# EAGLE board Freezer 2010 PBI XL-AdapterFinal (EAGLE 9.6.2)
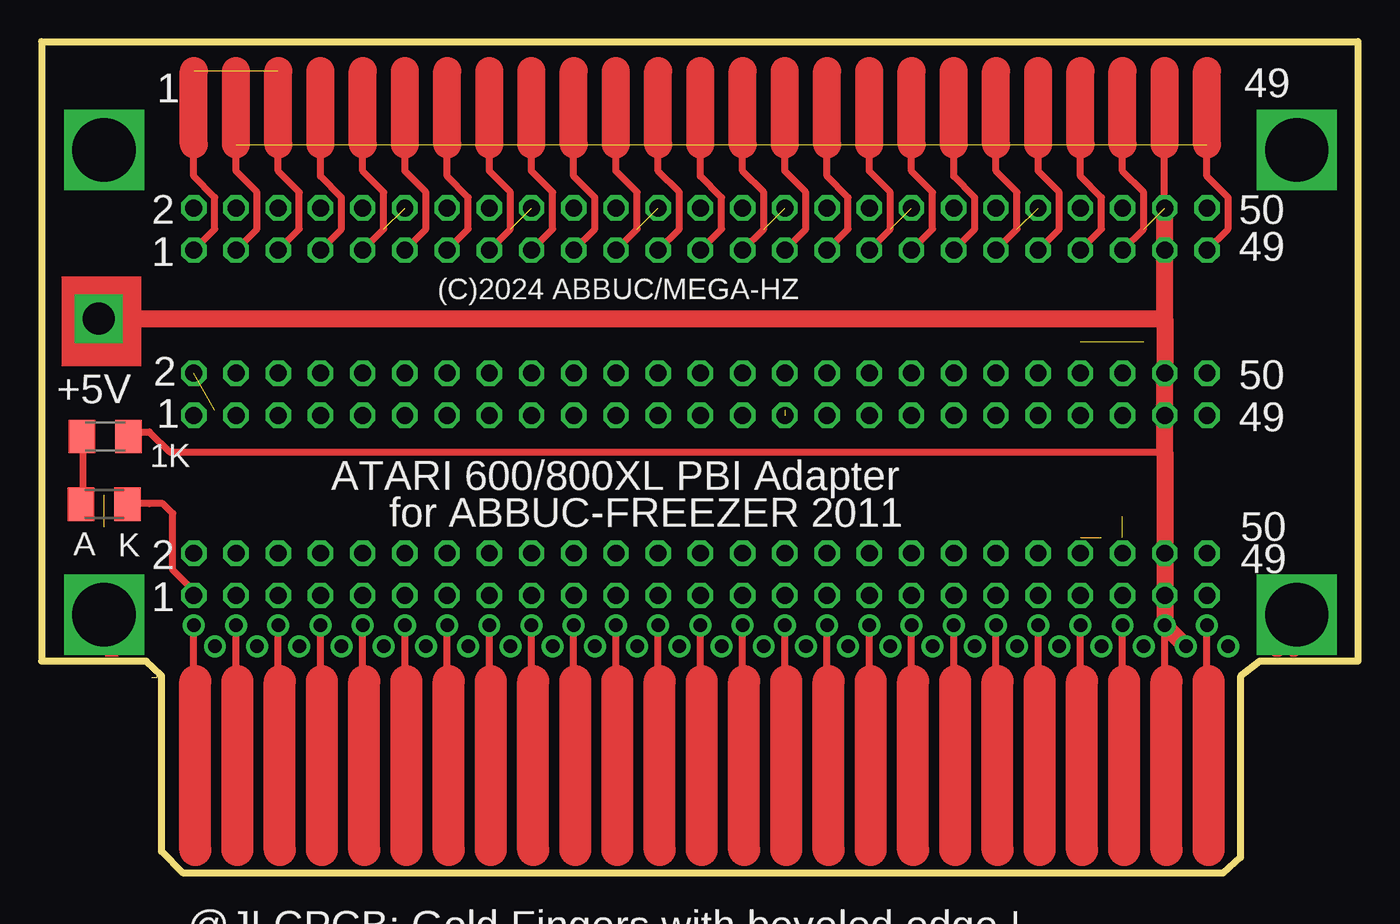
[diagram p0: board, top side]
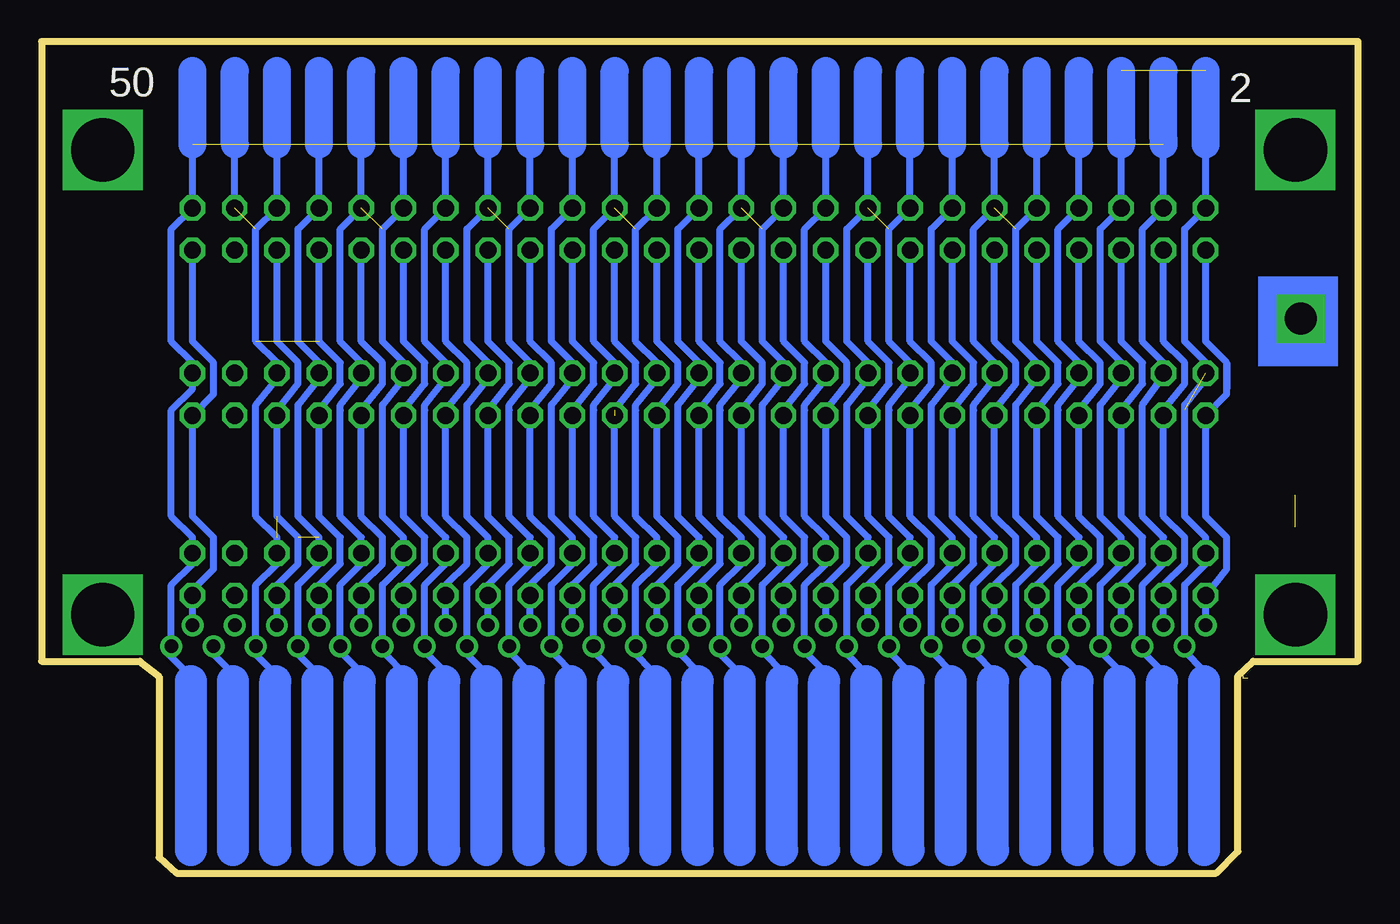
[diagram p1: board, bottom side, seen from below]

Size 79.2 x 50.05 mm. Coordinates in mm from the lower left corner, seen from the top.
Outline: 79.2,12.75 73.3,12.75 72.13,11.83 72.13,0.95 71.07,0 8.53,0 7.22,1.31 7.22,11.88 6.3,12.75 0,12.75 0,50.05 79.2,50.05 79.2,12.75
Copper layers (1*16): Top 0.035mm / dielectric 1.5mm / Bottom 0.035mm
Design rules "ITead_rule": minimum track width 6mil, minimum drill 12mil, track to track 6mil, track to pad 6mil, pad to pad 6mil, via to via 6mil, smd to smd 0mil, copper to edge 10mil, drill to drill 10mil, minimum pad ring 10mil, minimum via ring 6mil, stop-mask expansion 2mil, vias tented up to drill 100mil, thermal gap 10mil
Net classes: 2 3.3: width 0.508 mm, clearance 0.254 mm

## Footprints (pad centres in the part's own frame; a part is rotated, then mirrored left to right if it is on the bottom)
M1206 = smd 1.6 x 2: 1 -1.4,0; 2 1.4,0
XL-PBI = drill 0.813: A0 31.115,-8.255; A1 29.845,-6.985; A2 28.575,-8.255; A3 27.305,-6.985; A4 26.035,-8.255; A5 24.765,-6.985; A6 23.495,-8.255; A7 20.955,-8.255; A8 19.685,-6.985; A9 18.415,-8.255; A10 17.145,-6.985; A11 15.875,-8.255; A12 14.605,-6.985; A13 13.335,-8.255; A14 12.065,-6.985; A15 9.525,-6.985; AUDIO -27.305,-8.255; CAS -17.145,-8.255; D0 8.255,-8.255; D1 6.985,-6.985; D2 5.715,-8.255; D3 4.445,-6.985; D4 3.175,-8.255; D5 1.905,-6.985; D6 0.635,-8.255; D7 -0.635,-6.985; EXT.B -13.335,-6.985; EXTSEL 32.385,-6.985; GND -28.575,-6.985; GND2 -18.415,-6.985; GND3 -5.715,-6.985; GND4 -3.175,-6.985; GND5 22.225,-6.985; GND6 33.655,-8.255; GND7 10.795,-8.255; GND8 -1.905,-8.255; GND9 -22.225,-8.255; IRQ -9.525,-8.255; MPD -19.685,-8.255; NC2 -6.985,-8.255; NC3 -12.065,-8.255; NC4 -14.605,-8.255; PHI2 -4.445,-8.255; RAS -20.955,-6.985; RDY -10.795,-6.985; REF -15.875,-6.985; RST -8.255,-6.985; RW -23.495,-6.985; VCC -24.765,-8.255; VCC1 -26.035,-6.985

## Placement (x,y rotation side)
E$2  [M1206]  3.82,26.29 0 top
E$3  [M1206]  3.77,22.21 180 top
U$3  XL-PBI  [XL-PBI]  42.81,6.67 180 top

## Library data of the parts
E$2 E$3 = rcl
U$3 = wf-atari

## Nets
N$1: U$3.EXTSEL
N$16: U$3.AUDIO
N$28: U$3.VCC U$3.VCC1
N$32: U$3.GND9
N$33: U$3.MPD
N$34: U$3.CAS
N$35: U$3.NC4
N$37: U$3.NC3
N$38: U$3.IRQ
N$48: U$3.NC2
N$81: U$3.PHI2
N$88: U$3.GND8
N$89: U$3.D6
N$90: U$3.D4
N$91: U$3.D2
N$92: U$3.D0
N$93: U$3.GND7
N$94: U$3.A13
N$95: U$3.A11
N$96: U$3.A9
N$97: U$3.A7
N$98: U$3.A6
N$99: U$3.A4
N$102: U$3.RW
N$103: U$3.RAS
N$104: U$3.GND2
N$105: U$3.REF
N$106: U$3.EXT.B
N$107: U$3.RDY
N$108: U$3.RST
N$109: U$3.GND3
N$110: U$3.GND4
N$111: U$3.D7
N$112: U$3.D5
N$113: U$3.D3
N$114: U$3.D1
N$115: U$3.A15
N$116: U$3.A14
N$117: U$3.A12
N$118: U$3.A10
N$119: U$3.A8
N$120: U$3.GND5
N$122: U$3.A5
N$126: U$3.A1 U$3.A3
N$159: U$3.GND6
N$190: U$3.GND
N$307: U$3.A2
N$354: U$3.A0

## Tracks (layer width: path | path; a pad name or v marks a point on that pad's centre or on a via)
N$1  (via drill 1.02)  (1 unrouted)
  Bottom 0.406: 9.16,46.7 9.16,40.03 10.43,38.76 10.43,32 9.16,30.72 v9.16,30.09 | 10.43,27.87 10.43,21.48 9.16,20.21 v9.16,19.25 9.16,18.62 10.43,17.35 U$3.EXTSEL
N$16  (via drill 1.02)
  Bottom 0.406: U$3.AUDIO v70.12,16.72 70.12,17.03 68.85,18.3 68.85,20.21 70.12,21.48 70.12,27.55 68.85,28.82 68.85,30.72 70.12,32 v70.12,37.49
N$23  (via drill 1.02)
  other vias: 70.12,40.03
N$28  (via drill 1.02)
  Top 0.406: 4.78,26.56 6.49,26.56 7.7,25.35 67.58,25.35 67.6,25.35
  Top 1.016: 67.58,26.91 67.58,25.35 v67.58,19.25 v67.58,16.72 U$3.VCC U$3.VCC1
N$29  (via drill 1.02, 1.93)
  Top 0.406: 67.58,43.52 67.58,43.4 67.55,43.73 67.55,40.46 67.58,37.49
  Top 1.016: v67.58,27.55 v67.58,30.09 67.58,33.36 | 4.08,33.36 3.13,33.36 | 4.08,33.36 67.58,33.36 | v3.44,33.36 4.08,33.36 | 67.58,33.36 67.58,37.49 v67.58,40.03
N$30  (via drill 1.02)
  other vias: 65.04,40.03
N$31  (via drill 1.02)
  other vias: 62.5,40.03
N$32  (via drill 1.02)
  Bottom 0.406: U$3.GND9 v65.04,16.72
N$33  (via drill 1.02)
  Bottom 0.406: U$3.MPD v62.5,16.72
N$34  (via drill 1.02)
  Bottom 0.406: U$3.CAS v59.96,16.72
N$35  (via drill 1.02)
  Bottom 0.406: U$3.NC4 v57.42,16.72
N$36  (via drill 1.02)
  other vias: 59.96,40.03
N$37  (via drill 1.02)
  Bottom 0.406: U$3.NC3 v54.88,16.72
N$38  (via drill 1.02)
  Bottom 0.406: U$3.IRQ v52.34,16.72
N$39  (via drill 1.02)
  other vias: 57.42,40.03
N$40  (via drill 1.02)
  other vias: 54.88,40.03
N$41  (via drill 1.02)
  other vias: 52.34,40.03
N$42  (via drill 1.02)
  other vias: 49.8,40.03
N$43  (via drill 1.02)
  other vias: 47.26,40.03
N$44  (via drill 1.02)
  other vias: 44.72,40.03
N$45  (via drill 1.02)
  other vias: 42.18,40.03
N$46  (via drill 1.02)
  other vias: 39.64,40.03
N$47  (via drill 1.02)
  other vias: 37.1,40.03
N$48  (via drill 1.02)
  Bottom 0.406: U$3.NC2 v49.8,16.72
N$49  (via drill 1.02)
  other vias: 34.56,40.03
N$50  (via drill 1.02)
  other vias: 32.02,40.03
N$51  (via drill 1.02)
  other vias: 29.48,40.03
N$52  (via drill 1.02)
  other vias: 26.94,40.03
N$53  (via drill 1.02)
  other vias: 24.4,40.03
N$54  (via drill 1.02)
  other vias: 21.86,40.03
N$55  (via drill 1.02)
  other vias: 19.32,40.03
N$56  (via drill 1.02)
  other vias: 16.78,40.03
N$58
  Top 0.406: 19.32,43.84 19.32,42.25 20.59,40.98 20.59,38.76 19.32,37.49
N$59
  Top 0.406: 16.78,37.49 18.05,38.76 18.05,40.66 16.78,41.94 16.78,43.84
N$60
  Top 0.406: 21.86,43.52 21.86,42.25 23.13,40.98 23.13,38.76 21.86,37.49
N$62
  Top 0.406: 26.94,43.84 26.94,42.25 28.21,40.98 28.21,38.76 26.94,37.49
N$63
  Top 0.406: 24.4,37.49 25.67,38.76 25.67,40.66 24.4,41.94 24.4,43.84
N$64
  Top 0.406: 29.48,43.52 29.48,42.25 30.75,40.98 30.75,38.76 29.48,37.49
N$66
  Top 0.406: 34.56,43.84 34.56,42.25 35.83,40.98 35.83,38.76 34.56,37.49
N$67
  Top 0.406: 32.02,37.49 33.29,38.76 33.29,40.66 32.02,41.94 32.02,43.84
N$68
  Top 0.406: 37.1,43.52 37.1,42.25 38.37,40.98 38.37,38.76 37.1,37.49
N$70
  Top 0.406: 42.18,43.84 42.18,42.25 43.45,40.98 43.45,38.76 42.18,37.49
N$71
  Top 0.406: 39.64,37.49 40.91,38.76 40.91,40.66 39.64,41.94 39.64,43.84
N$72
  Top 0.406: 44.72,43.52 44.72,42.25 45.99,40.98 45.99,38.76 44.72,37.49
N$74
  Top 0.406: 49.8,43.84 49.8,42.25 51.07,40.98 51.07,38.76 49.8,37.49
N$75
  Top 0.406: 47.26,37.49 48.53,38.76 48.53,40.66 47.26,41.94 47.26,43.84
N$76
  Top 0.406: 52.34,43.52 52.34,42.25 53.61,40.98 53.61,38.76 52.34,37.49
N$78
  Top 0.406: 57.42,43.84 57.42,42.25 58.69,40.98 58.69,38.76 57.42,37.49
N$80
  Top 0.406: 54.88,37.49 56.15,38.76 56.15,40.66 54.88,41.94 54.88,43.84
N$81  (via drill 1.02)
  Bottom 0.406: U$3.PHI2 v47.26,16.72
N$82
  Top 0.406: 59.96,43.52 59.96,42.25 61.23,40.98 61.23,38.76 59.96,37.49
N$84
  Top 0.406: 65.04,43.84 65.04,42.25 66.31,40.98 66.31,38.76 65.04,37.49
N$85
  Top 0.406: 62.5,37.49 63.77,38.76 63.77,40.66 62.5,41.94 62.5,43.84
N$87
  Top 0.406: 70.12,37.49 71.39,38.76 71.39,40.66 70.12,41.94 70.12,43.84
N$88  (via drill 1.02)
  Bottom 0.406: U$3.GND8 v44.72,16.72
N$89  (via drill 1.02)
  Bottom 0.406: U$3.D6 v42.18,16.72
N$90  (via drill 1.02)
  Bottom 0.406: U$3.D4 v39.64,16.72
N$91  (via drill 1.02)
  Bottom 0.406: U$3.D2 v37.1,16.72
N$92  (via drill 1.02)
  Bottom 0.406: U$3.D0 v34.56,16.72
N$93  (via drill 1.02)
  Bottom 0.406: U$3.GND7 v32.02,16.72
N$94  (via drill 1.02)
  Bottom 0.406: U$3.A13 v29.48,16.72
N$95  (via drill 1.02)
  Bottom 0.406: U$3.A11 v26.94,16.72
N$96  (via drill 1.02)
  Bottom 0.406: U$3.A9 v24.4,16.72
N$97  (via drill 1.02)
  Bottom 0.406: U$3.A7 v21.86,16.72
N$98  (via drill 1.02)
  Bottom 0.406: U$3.A6 v19.32,16.72
N$99  (via drill 1.02)
  Bottom 0.406: U$3.A4 v16.78,16.72 16.78,17.35 15.51,18.62 15.51,20.21 16.78,21.48 16.78,27.87 15.51,29.45 15.51,30.72 16.78,32 v16.78,37.49
N$102
  Bottom 0.406: U$3.RW 66.31,17.35
N$103
  Bottom 0.406: U$3.RAS 63.77,17.35
N$104
  Bottom 0.406: U$3.GND2 61.23,17.35
N$105
  Bottom 0.406: U$3.REF 58.69,17.35
N$106
  Bottom 0.406: U$3.EXT.B 56.15,17.35
N$107
  Bottom 0.406: U$3.RDY 53.61,17.35
N$108
  Bottom 0.406: U$3.RST 51.07,17.35
N$109
  Bottom 0.406: U$3.GND3 48.53,17.35
N$110
  Bottom 0.406: U$3.GND4 45.99,17.35
N$111
  Bottom 0.406: U$3.D7 43.45,17.35
N$112
  Bottom 0.406: U$3.D5 40.91,17.35
N$113
  Bottom 0.406: U$3.D3 38.37,17.35
N$114
  Bottom 0.406: U$3.D1 35.83,17.35
N$115
  Bottom 0.406: U$3.A15 33.29,17.35
N$116
  Bottom 0.406: U$3.A14 30.75,17.35
N$117
  Bottom 0.406: U$3.A12 28.21,17.35
N$118
  Bottom 0.406: U$3.A10 25.67,17.35
N$119
  Bottom 0.406: U$3.A8 23.13,17.35
N$120
  Bottom 0.406: U$3.GND5 20.59,17.35
N$122
  Bottom 0.406: U$3.A5 18.05,17.35
N$123
  Bottom 0.406: 18.05,13.65 18.05,17.35 16.78,18.62 16.78,20.21 18.05,21.48
N$125
  Bottom 0.406: 20.59,13.65 20.59,17.35 19.32,18.62 19.32,20.21 20.59,21.48
N$126  (via drill 1.02)  (23 unrouted)
  Bottom 0.406: U$3.A1 12.97,17.35 11.7,18.62 v11.7,19.25 11.7,20.21 12.97,21.48 12.97,28.18 11.68,29.94 11.7,30.72 12.97,32 12.97,38.76 v11.7,40.03 11.7,44.16 | 14.24,44.16 v14.24,40.03 15.51,38.76 15.51,32 14.24,30.72 14.24,29.77 15.51,28.18 15.51,21.48 14.24,20.21 v14.24,19.25 14.24,18.62 15.51,17.35 U$3.A3
  Bottom 1.676: 70.12,43.84 70.12,48.28 | 67.58,43.84 67.58,48.28 | 65.04,43.84 65.04,48.28 | 62.5,43.84 62.5,48.28 | 59.96,43.84 59.96,48.28 | 57.42,43.84 57.42,48.28 | 54.88,43.84 54.88,48.28 | 52.34,43.84 52.34,48.28 | 49.8,43.84 49.8,48.28 | 47.26,43.84 47.26,48.28 | 44.72,43.84 44.72,48.28 | 42.18,43.84 42.18,48.28 | 39.64,43.84 39.64,48.28 | 37.1,43.84 37.1,48.28 | 34.56,43.84 34.56,48.28 | 32.02,43.84 32.02,48.28 | 29.48,43.84 29.48,48.28 | 26.94,43.84 26.94,48.28 | 24.4,43.84 24.4,48.28 | 21.86,43.84 21.86,48.28 | 19.32,43.84 19.32,48.28 | 16.78,43.84 16.78,48.28 | 11.7,43.84 11.7,44.16 11.7,48.28 | 14.24,43.84 14.24,44.16 14.24,48.28
N$129
  Bottom 0.406: 23.13,13.65 23.13,17.35 21.86,18.62 21.86,20.21 23.13,21.48
N$130
  Bottom 0.406: 25.67,13.65 25.67,17.35 24.4,18.62 24.4,20.21 25.67,21.48
N$132  (via drill 1.02)
  Bottom 0.406: 29.48,16.72 29.48,17.35 28.21,18.62 28.21,20.21 29.48,21.48 29.48,27.87 28.21,29.45 28.21,30.72 29.48,32 v29.48,37.49
N$133
  Bottom 0.406: 28.21,13.65 28.21,17.35 26.94,18.62 26.94,20.21 28.21,21.48
N$134
  Bottom 0.406: 30.75,13.65 30.75,17.35 29.48,18.62 29.48,20.21 30.75,21.48
N$137
  Bottom 0.406: 33.29,13.65 33.29,17.35 32.02,18.62 32.02,20.21 33.29,21.48
N$138
  Bottom 0.406: 35.83,13.65 35.83,17.35 34.56,18.62 34.56,20.21 35.83,21.48
N$140  (via drill 1.02)
  Bottom 0.406: 39.64,16.72 39.64,17.35 38.37,18.62 38.37,20.21 39.64,21.48 39.64,27.87 38.37,29.45 38.37,30.72 39.64,32 v39.64,37.49
N$141
  Bottom 0.406: 38.37,13.65 38.37,17.35 37.1,18.62 37.1,20.21 38.37,21.48
N$142
  Bottom 0.406: 40.91,13.65 40.91,17.35 39.64,18.62 39.64,20.21 40.91,21.48
N$144  (via drill 1.02)  (1 unrouted)
  Bottom 0.406: 44.72,16.72 44.72,17.35 43.45,18.62 43.45,20.21 44.72,21.48 44.72,27.87 43.45,29.45 43.45,30.72 44.72,32 v44.72,37.49
  other vias: 44.72,27.55
N$145
  Bottom 0.406: 43.45,13.65 43.45,17.35 42.18,18.62 42.18,20.21 43.45,21.48
N$146
  Bottom 0.406: 45.99,13.65 45.99,17.35 44.72,18.62 44.72,20.21 45.99,21.48
N$148  (via drill 1.02)
  Bottom 0.406: 49.8,16.72 49.8,17.35 48.53,18.62 48.53,20.21 49.8,21.48 49.8,27.87 48.53,29.45 48.53,30.72 49.8,32 v49.8,37.49
N$149
  Bottom 0.406: 48.53,13.65 48.53,17.35 47.26,18.62 47.26,20.21 48.53,21.48
N$150
  Bottom 0.406: 51.07,13.65 51.07,17.35 49.8,18.62 49.8,20.21 51.07,21.48
N$152  (via drill 1.02)
  Bottom 0.406: 54.88,16.72 54.88,17.35 53.61,18.62 53.61,20.21 54.88,21.48 54.88,27.87 53.61,29.45 53.61,30.72 54.88,32 v54.88,37.49
N$153
  Bottom 0.406: 53.61,13.65 53.61,17.35 52.34,18.62 52.34,20.21 53.61,21.48
N$154
  Bottom 0.406: 56.15,13.65 56.15,17.35 54.88,18.62 54.88,20.21 56.15,21.48
N$156  (via drill 1.02)
  Bottom 0.406: 59.96,16.72 59.96,17.35 58.69,18.62 58.69,20.21 59.96,21.48 59.96,27.87 58.69,29.45 58.69,30.72 59.96,32 v59.96,37.49
N$157
  Bottom 0.406: 58.69,13.65 58.69,17.35 57.42,18.62 57.42,20.21 58.69,21.48
N$158
  Bottom 0.406: 61.23,13.65 61.23,17.35 59.96,18.62 59.96,20.21 61.23,21.48
N$159  (via drill 1.02)  (23 unrouted)
  Top 0.406: v9.16,37.49 10.43,38.76 10.43,40.66 9.16,41.94 9.16,43.84 | v9.16,16.72 9.16,16.99 7.9,18.25 7.9,21.65 7.3,22.25 6.5,22.25 5.2,22.25
  Top 1.676: 9.16,43.84 9.16,48.28 | 14.24,43.84 14.24,48.28 | 16.78,43.84 16.78,48.28 | 19.32,43.84 19.32,48.28 | 21.86,43.84 21.86,48.28 | 24.4,43.84 24.4,48.28 | 26.94,43.84 26.94,48.28 | 29.48,43.84 29.48,48.28 | 32.02,43.84 32.02,48.28 | 34.56,43.84 34.56,48.28 | 37.1,43.84 37.1,48.28 | 39.64,43.84 39.64,48.28 | 42.18,43.84 42.18,48.28 | 44.72,43.84 44.72,48.28 | 47.26,43.84 47.26,48.28 | 49.8,43.84 49.8,48.28 | 52.34,43.84 52.34,48.28 | 54.88,43.84 54.88,48.28 | 57.42,43.84 57.42,48.28 | 59.96,43.84 59.96,48.28 | 62.5,43.84 62.5,48.28 | 65.04,43.84 65.04,48.28 | 67.58,43.84 67.58,48.28 | 70.12,43.84 70.12,48.28
  Bottom 0.406: 9.16,32 9.16,37.17 | 7.89,30.72 7.89,29.14 | 9.16,26.96 9.16,27.19 | 9.16,32 v9.16,37.49 | 7.89,30.72 9.16,32 | 7.89,30.72 7.89,28.82 v9.16,27.55 9.16,26.96 | 9.16,26.96 9.16,21.48 7.89,20.21 7.89,18.3 v9.16,16.72 U$3.GND6
N$160
  Bottom 0.406: 11.7,27.23 11.7,27.87 10.43,29.45 10.43,30.72 11.7,32 11.7,37.17
N$162
  Top 1.016: 67.58,27.23 67.58,29.77
N$166
  Bottom 0.406: 10.43,38.44 10.43,32 9.16,30.72 9.16,29.77 10.43,28.18 10.43,25.92
N$169
  Bottom 0.406: 18.05,21.48 18.05,27.87
N$170
  Bottom 0.406: 20.59,21.48 20.59,27.87
N$171
  Bottom 0.406: 23.13,21.48 23.13,27.87
N$172
  Bottom 0.406: 25.67,21.48 25.67,27.87
N$173
  Bottom 0.406: 28.21,21.48 28.21,27.87
N$174
  Bottom 0.406: 30.75,21.48 30.75,27.87
N$175
  Bottom 0.406: 33.29,21.48 33.29,27.87
N$176
  Bottom 0.406: 35.83,21.48 35.83,27.87
N$177
  Bottom 0.406: 38.37,21.48 38.37,27.87
N$178
  Bottom 0.406: 40.91,21.48 40.91,27.87
N$179
  Bottom 0.406: 43.45,21.48 43.45,27.87
N$180
  Bottom 0.406: 45.99,21.48 45.99,27.87
N$181
  Bottom 0.406: 48.53,21.48 48.53,27.87
N$182  (via drill 1.02)
  other vias: 11.7,30.09
N$183
  Bottom 0.406: 51.07,21.48 51.07,27.87
N$184
  Bottom 0.406: 66.31,21.48 66.31,28.18
N$185
  Bottom 0.406: 63.77,21.48 63.77,28.18
N$186
  Bottom 0.406: 61.23,21.48 61.23,27.87
N$187
  Bottom 0.406: 58.69,21.48 58.69,27.87
N$188
  Bottom 0.406: 56.15,21.48 56.15,27.87
N$189
  Bottom 0.406: 53.61,21.48 53.61,27.87
N$190
  Bottom 0.406: U$3.GND 71.39,17.35 70.12,18.62 70.12,20.21 71.39,21.48 71.39,27.87 70.12,29.14 70.12,30.72 71.39,32 71.39,38.76 70.12,40.03 70.12,46.7
N$191  (via drill 1.02)
  Bottom 0.406: 21.86,16.72 21.86,17.35 20.59,18.62 20.59,20.21 21.86,21.48 21.86,27.87 20.59,29.45 20.59,30.72 21.86,32 v21.86,37.49
N$193
  Bottom 0.406: 18.05,21.48 18.05,28.18 16.78,29.77 16.78,30.72 18.05,32 18.05,38.76 16.78,40.03 16.78,46.7
N$195  (via drill 1.02)
  Bottom 0.406: 26.94,16.72 26.94,17.35 25.67,18.62 25.67,20.21 26.94,21.48 26.94,27.87 25.67,29.45 25.67,30.72 26.94,32 v26.94,37.49
N$197  (1 unrouted)
  Bottom 0.406: 23.13,21.48 23.13,28.18 21.86,29.77 21.86,30.72 23.13,32 23.13,38.76 21.86,40.03 21.86,44.16 | 20.59,21.48 20.59,28.18 19.32,29.77 19.32,30.72 20.59,32 20.59,38.76 19.32,40.03 19.32,44.16
N$198
  Bottom 0.406: 25.67,21.48 25.67,28.18 24.4,29.77 24.4,30.72 25.67,32 25.67,38.76 24.4,40.03 24.4,46.7
N$199  (via drill 1.02)
  Bottom 0.406: 32.02,16.72 32.02,17.35 30.75,18.62 30.75,20.21 32.02,21.48 32.02,27.87 30.75,29.45 30.75,30.72 32.02,32 v32.02,37.49
N$202  (1 unrouted)
  Bottom 0.406: 30.75,21.48 30.75,28.18 29.48,29.77 29.48,30.72 30.75,32 30.75,38.76 29.48,40.03 29.48,44.16 | 28.21,21.48 28.21,28.18 26.94,29.77 26.94,30.72 28.21,32 28.21,38.76 26.94,40.03 26.94,44.16
N$203  (via drill 1.02)
  Bottom 0.406: 37.1,16.72 37.1,17.35 35.83,18.62 35.83,20.21 37.1,21.48 37.1,27.87 35.83,29.45 35.83,30.72 37.1,32 v37.1,37.49
N$204  (via drill 1.02)
  Bottom 0.406: 34.56,16.72 34.56,17.35 33.29,18.62 33.29,20.21 34.56,21.48 34.56,27.87 33.29,29.45 33.29,30.72 34.56,32 v34.56,37.49
N$205
  Bottom 0.406: 33.29,21.48 33.29,28.18 32.02,29.77 32.02,30.72 33.29,32 33.29,38.76 32.02,40.03 32.02,46.7
N$207  (via drill 1.02)
  Bottom 0.406: 42.18,16.72 42.18,17.35 40.91,18.62 40.91,20.21 42.18,21.48 42.18,27.87 40.91,29.45 40.91,30.72 42.18,32 v42.18,37.49
N$209  (1 unrouted)
  Bottom 0.406: 38.37,21.48 38.37,28.18 37.1,29.77 37.1,30.72 38.37,32 38.37,38.76 37.1,40.03 37.1,44.16 | 35.83,21.48 35.83,28.18 34.56,29.77 34.56,30.72 35.83,32 35.83,38.76 34.56,40.03 34.56,44.16
N$210
  Bottom 0.406: 40.91,21.48 40.91,28.18 39.64,29.77 39.64,30.72 40.91,32 40.91,38.76 39.64,40.03 39.64,46.7
N$211  (via drill 1.02)
  Bottom 0.406: 47.26,16.72 47.26,17.35 45.99,18.62 45.99,20.21 47.26,21.48 47.26,27.87 45.99,29.45 45.99,30.72 47.26,32 v47.26,37.49
N$214  (1 unrouted)
  Bottom 0.406: 45.99,21.48 45.99,28.18 44.72,29.77 44.72,30.72 45.99,32 45.99,38.76 44.72,40.03 44.72,44.16 | 43.45,21.48 43.45,28.18 42.18,29.77 42.18,30.72 43.45,32 43.45,38.76 42.18,40.03 42.18,44.16
N$215  (via drill 1.02)
  Bottom 0.406: 52.34,16.72 52.34,17.35 51.07,18.62 51.07,20.21 52.34,21.48 52.34,27.87 51.07,29.45 51.07,30.72 52.34,32 v52.34,37.49
N$217
  Bottom 0.406: 48.53,21.48 48.53,28.18 46.94,30.09 47.26,30.72 48.53,32 48.53,38.76 47.26,40.03 47.26,46.7
N$219  (via drill 1.02)
  Bottom 0.406: 57.42,27.55 57.42,27.23 | 57.42,27.55 57.42,27.87 56.15,29.45 56.15,30.72 57.42,32 v57.42,37.49 | 57.42,16.72 57.42,17.35 56.15,18.62 56.15,20.21 57.42,21.48 57.42,27.55
N$221  (1 unrouted)
  Bottom 0.406: 53.61,21.48 53.61,28.18 52.34,29.77 52.34,30.72 53.61,32 53.61,38.76 52.34,40.03 52.34,44.16 | 51.07,21.48 51.07,28.18 49.8,29.77 49.8,30.72 51.07,32 51.07,38.76 49.8,40.03 49.8,44.16
N$222
  Bottom 0.406: 56.15,21.48 56.15,28.18 54.88,29.77 54.88,30.72 56.15,32 56.15,38.76 54.88,40.03 54.88,46.7
N$223  (via drill 1.02)  (6 unrouted)
  Bottom 0.406: 63.77,28.18 62.5,29.77 62.5,30.72 63.77,32 63.77,38.76 62.5,40.03 62.5,46.7 | 66.31,28.18 65.04,29.77 65.04,30.72 66.31,32 66.31,38.76 65.04,40.03 65.04,44.16 | 62.5,16.72 62.5,17.35 61.23,18.62 61.23,20.21 62.5,21.48 62.5,27.87 61.23,29.45 61.23,30.72 62.5,32 v62.5,37.49 | 63.77,17.35 62.5,18.62 62.5,20.21 63.77,21.48 | 65.04,17.35 63.77,18.62 63.77,20.21 65.04,21.48 65.04,27.87 63.77,29.45 63.77,30.72 65.04,32 v65.04,37.49 | 66.31,17.35 65.04,18.62 65.04,20.21 66.31,21.48 | 67.58,40.03 67.58,44.16
N$226  (1 unrouted)
  Bottom 0.406: 61.23,21.48 61.23,28.18 59.96,29.77 59.96,30.72 61.23,32 61.23,38.76 59.96,40.03 59.96,44.16 | 58.69,21.48 58.69,28.18 57.42,29.77 57.42,30.72 58.69,32 58.69,38.76 57.42,40.03 57.42,44.16
N$231  (via drill 3.81)
  other vias: 3.76,43.52
N$232  (via drill 3.81)
  other vias: 75.52,43.52
N$233  (via drill 3.81)
  other vias: 75.52,15.56
N$234  (via drill 3.81)
  other vias: 3.76,15.56
N$284  (via drill 1.02)
  other vias: 67.58,37.49
N$301  (via drill 1.02)
  Bottom 0.406: 24.4,16.72 24.4,17.35 23.13,18.62 23.13,20.21 24.4,21.48 24.4,27.55 | 24.4,27.55 24.4,27.23 | 24.4,27.55 24.4,27.87 23.13,29.45 23.13,30.72 24.4,32 v24.4,37.49
N$303  (via drill 1.02)
  Bottom 0.406: 19.32,16.72 19.32,17.35 18.05,18.62 18.05,20.21 19.32,21.48 19.32,27.87 18.05,29.45 18.05,30.72 19.32,32 v19.32,37.49
N$304  (via drill 1.02)
  Top 0.406: 11.7,43.84 11.7,42.25 12.97,40.98 12.97,38.76 v11.7,37.49
  Top 1.676: 11.7,43.84 11.7,48.28
N$307  (via drill 1.02)
  Top 0.406: 14.24,43.52 14.24,42.25 15.51,40.98 15.51,38.76 v14.24,37.49
  Bottom 0.406: 14.24,37.17 v14.24,37.49 14.24,32 12.97,30.72 12.97,29.45 14.24,27.87 14.24,27.55 | U$3.A2 v14.24,16.72 14.24,17.35 12.97,18.62 12.97,20.21 14.24,21.48 14.24,27.55 | 14.24,27.55 14.24,27.23
N$308  (via drill 1.02)
  other vias: 70.12,27.55
N$310  (via drill 1.02)
  other vias: 65.04,27.55
N$311  (via drill 1.02)
  other vias: 62.5,27.55
N$312  (via drill 1.02)
  other vias: 59.96,27.55
N$313  (via drill 1.02)
  other vias: 57.42,27.55
N$314  (via drill 1.02)
  other vias: 54.88,27.55
N$315  (via drill 1.02)
  other vias: 52.34,27.55
N$316  (via drill 1.02)
  other vias: 49.8,27.55
N$317  (via drill 1.02)
  other vias: 47.26,27.55
N$319  (via drill 1.02)
  other vias: 42.18,27.55
N$320  (via drill 1.02)
  other vias: 39.64,27.55
N$321  (via drill 1.02)
  other vias: 37.1,27.55
N$322  (via drill 1.02)
  other vias: 34.56,27.55
N$323  (via drill 1.02)
  other vias: 32.02,27.55
N$324  (via drill 1.02)
  other vias: 29.48,27.55
N$325  (via drill 1.02)
  other vias: 26.94,27.55
N$326  (via drill 1.02)
  other vias: 24.4,27.55
N$327  (via drill 1.02)
  other vias: 21.86,27.55
N$328  (via drill 1.02)
  other vias: 19.32,27.55
N$330  (via drill 1.02)
  other vias: 16.78,27.55
N$332  (via drill 1.02)
  other vias: 14.24,27.55
N$333  (via drill 1.02)
  other vias: 70.12,30.09
N$335  (via drill 1.02)
  other vias: 65.04,30.09
N$336  (via drill 1.02)
  other vias: 62.5,30.09
N$337  (via drill 1.02)
  other vias: 59.96,30.09
N$338  (via drill 1.02)
  other vias: 57.42,30.09
N$339  (via drill 1.02)
  other vias: 54.88,30.09
N$340  (via drill 1.02)
  other vias: 52.34,30.09
N$341  (via drill 1.02)
  other vias: 49.8,30.09
N$342  (via drill 1.02)
  other vias: 47.26,30.09
N$343  (via drill 1.02)
  other vias: 44.72,30.09
N$344  (via drill 1.02)
  other vias: 42.18,30.09
N$345  (via drill 1.02)
  other vias: 39.64,30.09
N$346  (via drill 1.02)
  other vias: 37.1,30.09
N$347  (via drill 1.02)
  other vias: 34.56,30.09
N$348  (via drill 1.02)
  other vias: 32.02,30.09
N$349  (via drill 1.02)
  other vias: 29.48,30.09
N$350  (via drill 1.02)
  other vias: 26.94,30.09
N$351  (via drill 1.02)
  other vias: 24.4,30.09
N$352  (via drill 1.02)
  other vias: 21.86,30.09
N$353  (via drill 1.02)
  other vias: 19.32,30.09
N$354  (via drill 1.02)
  Bottom 0.406: U$3.A0 v11.7,16.72 11.7,17.35 10.43,18.62 10.43,20.21 11.7,21.48 v11.7,27.55
N$355  (via drill 1.02)
  other vias: 16.78,30.09
N$357  (via drill 1.02)
  other vias: 14.24,30.09
S$1  (1 unrouted)
S$2
  Top 0.406: 2.5,22.35 2.5,26.25
S$3
  Bottom 1.676: 9.16,43.84 9.16,48.28
S$6  (via drill 1.02)
  other vias: 9.16,40.03
S$8  (via drill 1.02)
  other vias: 16.78,19.25
S$9  (via drill 1.02)
  other vias: 19.32,19.25
S$11  (via drill 1.02)
  other vias: 21.86,19.25
S$13  (via drill 1.02)
  other vias: 24.4,19.25
S$15  (via drill 1.02)
  other vias: 26.94,19.25
S$17  (via drill 1.02)
  other vias: 29.48,19.25
S$19  (via drill 1.02)
  other vias: 32.02,19.25
S$21  (via drill 1.02)
  other vias: 34.56,19.25
S$23  (via drill 1.02)
  other vias: 37.1,19.25
S$24  (via drill 1.02)
  other vias: 39.64,19.25
S$25  (via drill 1.02)
  other vias: 42.18,19.25
S$26  (via drill 1.02)
  other vias: 44.72,19.25
S$27  (via drill 1.02)
  other vias: 47.26,19.25
S$28  (via drill 1.02)
  other vias: 49.8,19.25
S$29  (via drill 1.02)
  other vias: 65.04,19.25
S$30  (via drill 1.02)
  other vias: 62.5,19.25
S$31  (via drill 1.02)
  other vias: 59.96,19.25
S$32  (via drill 1.02)
  other vias: 57.42,19.25
S$33  (via drill 1.02)
  other vias: 54.88,19.25
S$34  (via drill 1.02)
  other vias: 52.34,19.25
S$35  (via drill 1.02)
  other vias: 70.12,19.25
S$56
  Top 0.406: 67.85,48.7 67.65,48.5
(copper drawn outside any net)
  shapes: Bottom area x1, Top area x1

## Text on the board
tPlace: 49 | 1 | 2 | 50 | 49 | 1 | (C)2024 ABBUC/MEGA-HZ | 2 | 50 | +5V | 1 | 49 | 1K | ATARI 600/800XL PBI Adapter | for ABBUC-FREEZER 2011 | 50 | A | K | 2 | 49 | 1 | @JLCPCB: Gold Fingers with beveled edge !
bPlace: 50 | 2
